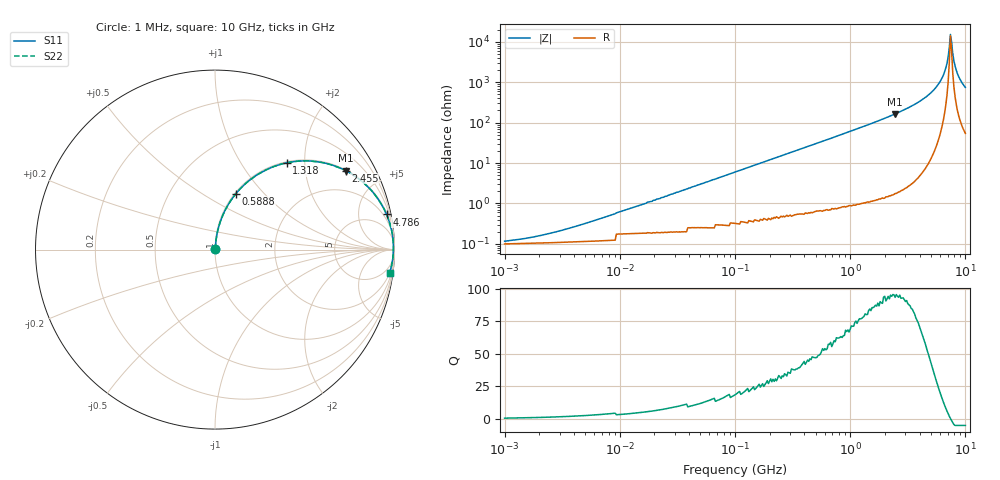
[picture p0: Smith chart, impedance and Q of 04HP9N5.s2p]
# MHz S MA R 50
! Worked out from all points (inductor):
!   401 points, 1 MHz to 10 GHz, reference 50 ohm
!   read as one part in series: L = 9.5 nH near 5.888 MHz
!   highest Q = 95 at 2.455 GHz (marker M1), where L = 10.7 nH
!   self-resonance near 7.413 GHz
!   S11 on the Smith chart (normalised r, x): 1 MHz: 1.00, +0.00; 588.8 MHz: 1.01, +0.71; 1.318 GHz: 1.02, +1.63; 2.455 GHz: 1.04, +3.29; 4.786 GHz: 1.18, +9.72; 10 GHz: 2, -15
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1  0.001157 31.0  0.999 -0.0  0.999 -0.0  0.001157 31.0
2.042  0.001638 47.9  0.999 -0.1  0.999 -0.1  0.001638 47.9
4.677  0.003066 65.3  0.999 -0.2  0.999 -0.2  0.003066 65.3
21.878  0.013 81.0  0.998 -0.7  0.998 -0.7  0.013 81.0
102.329  0.061 83.5  0.995 -3.5  0.995 -3.5  0.061 83.5
467.735  0.268 73.2  0.958 -15.6  0.958 -15.6  0.268 73.2
588.844  0.332 69.6  0.937 -19.4  0.937 -19.4  0.332 69.6
1318.257  0.627 50.5  0.771 -38.8  0.771 -38.8  0.627 50.5
2187.762  0.815 34.8  0.57 -54.6  0.57 -54.6  0.815 34.8
2454.709  0.85 31.2  0.517 -58.2  0.517 -58.2  0.85 31.2
3548.134  0.936 20.0  0.342 -69.3  0.342 -69.3  0.936 20.0
4786.301  0.976 11.6  0.201 -77.3  0.201 -77.3  0.976 11.6
5623.413  0.987 7.3  0.127 -80.7  0.127 -80.7  0.987 7.3
6309.573  0.992 4.3  0.075 -81.9  0.075 -81.9  0.992 4.3
6760.83  0.994 2.5  0.044 -80.5  0.044 -80.5  0.994 2.5
7244.36  0.994 0.7  0.014 -64.7  0.014 -64.7  0.994 0.7
7413.102  0.994 0.1  0.00653 -22.5  0.00653 -22.5  0.994 0.1
7762.471  0.993 -1.0  0.019 69.3  0.019 69.3  0.993 -1.0
8128.305  0.992 -2.2  0.039 77.7  0.039 77.7  0.992 -2.2
8511.38  0.991 -3.4  0.06 79.5  0.06 79.5  0.991 -3.4
9120.108  0.988 -5.2  0.09 79.6  0.09 79.6  0.988 -5.2
10000  0.982 -7.5  0.132 78.3  0.132 78.3  0.982 -7.5
